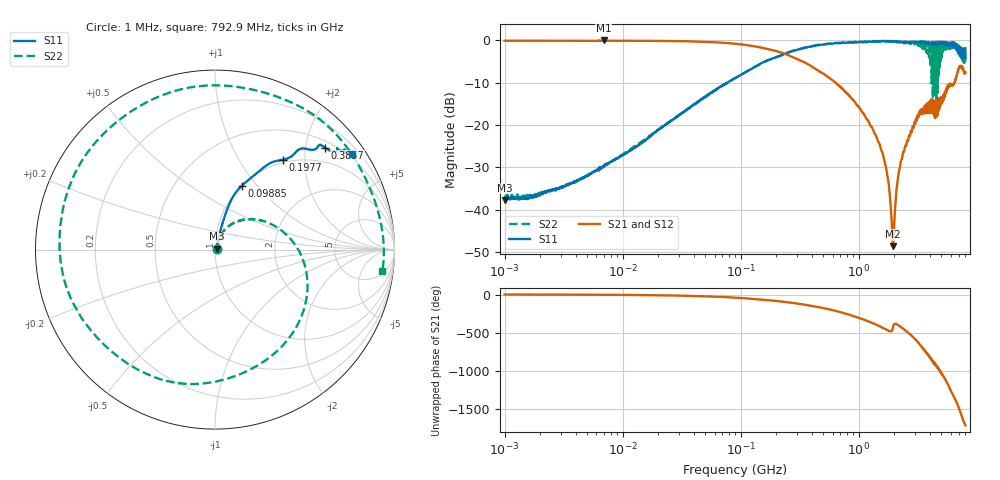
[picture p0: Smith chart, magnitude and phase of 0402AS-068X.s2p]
!s-Parameter Generated by FASTRON Sdn. Bhd.
!FASTRON P/N : 0402AS-068X
!Keysight Technologies: E5071C_MY46733604_B.14.02
!Date: Mon Dec 01 10:48:06 2025
!Version  :Rev00  Mon Dec 01 10:48:06 2025
!Data & Calibration Information:
!Freq  S11:SOLT2(ON)  S21:SOLT2(ON)  S12:SOLT2(ON)  S22:SOLT2(ON)
!PortZ  Port1:50+j0  Port2:50+j0
!When reading reference impedance value at option line is always used.
! Remarks : This data is being provided solely for informational purposes.
# Hz S dB R 50
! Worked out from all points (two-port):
!   1601 points, 1 MHz to 8 GHz, reference 50 ohm
!   highest |S21| = -0.05 dB at 6.912 MHz (marker M1); lowest = -48.6 dB at 1.944 GHz (marker M2)
!   |S21| within 3 dB of the highest: start of sweep to 228.9 MHz
!   lowest |S11| = -37.7 dB at 1.007 MHz (marker M3), VSWR 1.03, Z = 51.2 + j0.472 ohm
!   |S11| at or under -10 dB: start of sweep to 76.55 MHz
!   |S22| runs from -37.7 to -0.2 dB; largest |S21 - S12| = 0.012
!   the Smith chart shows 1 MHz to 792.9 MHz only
!   S11 on the Smith chart (normalised r, x): 1 MHz: 1.03, +0.01; 98.85 MHz: 1.00, +0.84; 197.7 MHz: 0.95, +1.57; 385.7 MHz: 0.64, +2.41; 792.9 MHz: 0.38, +3.14
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1000000  -37.30 21.4  -0.11 -0.5  -0.12 -0.5  -36.90 19.3
1006601  -37.70 20.7  -0.12 -0.5  -0.12 -0.6  -37.00 20.0
4479405  -32.70 55.7  -0.13 -2.2  -0.12 -2.2  -32.70 54.9
6911657  -29.70 60.3  -0.05 -3.4  -0.10 -3.2  -29.60 58.6
2.00676e7  -21.20 74.4  -0.17 -9.6  -0.17 -9.6  -21.10 67.2
8.994653e7  -8.91 68.9  -0.83 -41.1  -0.82 -41.1  -8.94 21.6
9.885233e7  -8.27 67.2  -0.94 -44.9  -0.94 -44.9  -8.27 16.0
1.976721e8  -4.04 52.9  -2.52 -83.4  -2.51 -83.4  -4.05 -44.3
3.856923e8  -1.56 42.7  -5.92 -146.0  -5.91 -146.0  -1.51 -157.0
4.006501e8  -1.47 40.9  -6.21 -150.0  -6.20 -150.0  -1.40 -164.0
7.929002e8  -0.61 34.9  -12.50 105.0  -12.50 105.0  -0.54 -7.3
1.120185e9  -0.29 39.8  -17.70 26.3  -17.70 26.2  -0.48 -172.0
1.334081e9  -0.24 46.1  -21.40 -21.4  -21.40 -21.6  -0.36 84.4
1.535164e9  -0.20 52.7  -25.50 -64.4  -25.50 -64.5  -0.28 -10.8
1.7949e9  -0.19 59.9  -34.00 -117.0  -34.10 -117.0  -0.36 -136.0
1.944035e9  -0.36 63.0  -48.60 -79.0  -48.90 -78.6  -0.21 154.0
2.237469e9  -0.47 69.1  -29.80 -57.6  -29.80 -57.6  -0.29 9.1
2.618947e9  -0.48 79.5  -23.60 -141.0  -23.60 -141.0  -0.34 -177.0
2.985754e9  -0.43 90.0  -19.60 135.0  -19.60 135.0  -0.70 -0.7
3.345355e9  -0.52 99.2  -16.40 48.3  -16.40 48.0  -1.55 -178.0
3.710194e9  -0.73 108.0  -16.00 -30.1  -16.00 -30.6  -0.32 18.7
8e9  -1.89 -107.0  -7.76 81.2  -7.79 80.9  -4.07 124.0
